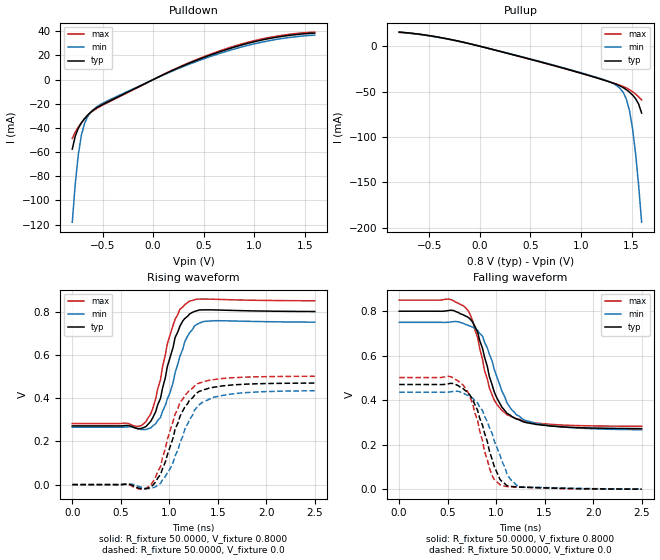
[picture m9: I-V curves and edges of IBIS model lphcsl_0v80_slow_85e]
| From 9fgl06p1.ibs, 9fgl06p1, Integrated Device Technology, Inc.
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[Model]   lphcsl_0v80_slow_85e
Model_type Output
Polarity   Inverting
Enable   Active-High
Vmeas =  0.4000V
Cref =   2.0000pF
Rref =   0.0
Vref =   0.4000V
C_comp   1.1000pF   1.0000pF   1.2000pF
[Temperature Range]   25.0000   85.0000   -40.0
[Voltage Range]   0.8000V   0.7500V   0.8500V
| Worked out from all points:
|   slope of the pulldown table from 0 to 0.12 V, typ, clamps not added: 24.7 ohm
|   slope of the pullup table from 0 to 0.12 V, typ, clamps not added: 35.2 ohm
|   rising waveform, R_fixture 50.0000, V_fixture 0.8000: 20-80 % time 187ps typ, 200ps min, 180ps max; typ from 0.272 V to 0.801 V
|   rising waveform, R_fixture 50.0000, V_fixture 0.0: 20-80 % time 242ps typ, 243ps min, 228ps max; typ from 0 V to 0.47 V
|   falling waveform, R_fixture 50.0000, V_fixture 0.8000: 20-80 % time 232ps typ, 262ps min, 217ps max; typ from 0.8 V to 0.272 V
|   falling waveform, R_fixture 50.0000, V_fixture 0.0: 20-80 % time 204ps typ, 234ps min, 186ps max; typ from 0.471 V to 0 V
[Pulldown]
|Voltage   I(typ)   I(min)   I(max)
-800mV    -57.5mA    -118mA     -48.67mA
-770mV    -46.59mA   -85.85mA   -43.39mA
-740mV    -40.19mA   -61.9mA    -39.31mA
-710mV    -35.84mA   -46.06mA   -35.76mA
-680mV    -32.42mA   -36.54mA   -32.6mA
-650mV    -29.55mA   -30.89mA   -29.85mA
-620mV    -27.13mA   -27.25mA   -27.51mA
-560mV    -23.38mA   -22.64mA   -23.91mA
130mV     5.245mA    4.902mA    5.439mA
640mV     22.49mA    21.15mA    23.23mA
1.12V     33.55mA    31.75mA    34.44mA
1.6V      38.53mA    36.86mA    39.36mA
[Pullup]
|Voltage   I(typ)   I(min)   I(max)
-800mV    15.6mA     15.6mA     15.19mA
-410mV    9.958mA    9.715mA    9.961mA
70mV      -1.984mA   -1.918mA   -2.008mA
1.03V     -30.65mA   -30.15mA   -30.73mA
1.36V     -42.39mA   -43.87mA   -42mA
1.42V     -45.75mA   -51.28mA   -44.47mA
1.45V     -47.95mA   -58.62mA   -46mA
1.48V     -50.57mA   -71.02mA   -47.85mA
1.51V     -53.7mA    -90.53mA   -50.08mA
1.54V     -57.7mA    -118mA     -52.7mA
1.57V     -63.58mA   -152.8mA   -55.69mA
1.6V      -73.58mA   -193.8mA   -59.07mA
[Ramp]
| variable   typ   min   max
dV/dt_r  0.2819/0.2350n   0.2606/0.2589n   0.3008/0.2225n
dV/dt_f  0.3166/0.2275n   0.2897/0.2556n   0.3403/0.2185n
R_load = 50.0000
[Rising Waveform]
R_fixture= 50.0000
V_fixture= 0.8000
V_fixture_min= 0.7500
V_fixture_max= 0.8500
|time   V(typ)   V(min)   V(max)
0s        271.6mV    265.6mV    282.5mV
680ps     258.9mV    257.8mV    269.5mV
760ps     268.9mV    255.2mV    291.7mV
830ps     309.7mV    271.4mV    352.5mV
910ps     399.6mV    311.3mV    486.4mV
980ps     546.4mV    396.3mV    651.9mV
1.06ns    680.7mV    517.2mV    764.5mV
1.21ns    789.9mV    702.9mV    849.5mV
1.36ns    808.7mV    755.2mV    858.6mV
2.5ns     801mV      751.6mV    850.7mV
[Rising Waveform]
R_fixture= 50.0000
V_fixture= 0.0
V_fixture_min= 0.0
V_fixture_max= 0.0
|time   V(typ)   V(min)   V(max)
0s        0V         0V         0V
610ps     -1.214mV   2.177mV    -4.958mV
780ps     -16.92mV   -17.96mV   -11mV
910ps     46.65mV    5.761mV    83.67mV
1.01ns    176.8mV    74.12mV    251.3mV
1.11ns    315.4mV    192.9mV    380.6mV
1.16ns    358.4mV    256.1mV    411.6mV
1.29ns    425.9mV    359.9mV    466.5mV
1.59ns    458.6mV    416.2mV    492.5mV
2.5ns     469.8mV    434.4mV    501.3mV
[Falling Waveform]
R_fixture= 50.0000
V_fixture= 0.8000
V_fixture_min= 0.7500
V_fixture_max= 0.8500
|time   V(typ)   V(min)   V(max)
0s        800mV      750mV      850mV
510ps     803.2mV    750.2mV    854.6mV
680ps     779.3mV    741.2mV    817.9mV
760ps     749.8mV    728.6mV    754.1mV
860ps     632.5mV    687.3mV    583.1mV
980ps     437.5mV    538.8mV    400.9mV
1.11ns    341.6mV    389.2mV    335.1mV
1.21ns    315.4mV    334mV      316.2mV
1.41ns    291.3mV    296mV      297.5mV
2.5ns     272.4mV    267.2mV    282.9mV
[Falling Waveform]
R_fixture= 50.0000
V_fixture= 0.0
V_fixture_min= 0.0
V_fixture_max= 0.0
|time   V(typ)   V(min)   V(max)
0s        470.6mV    436mV      501.8mV
510ps     474mV      436.1mV    507.3mV
660ps     452mV      432.5mV    468.1mV
760ps     402.4mV    408.3mV    380.4mV
860ps     287mV      353.5mV    216.9mV
960ps     132.6mV    248.9mV    60.3mV
1.06ns    34.31mV    125.6mV    15.41mV
1.14ns    13.7mV     48.96mV    10.62mV
1.24ns    9.537mV    11.91mV    9.449mV
2.5ns     378uV      802.6uV    220.9uV
